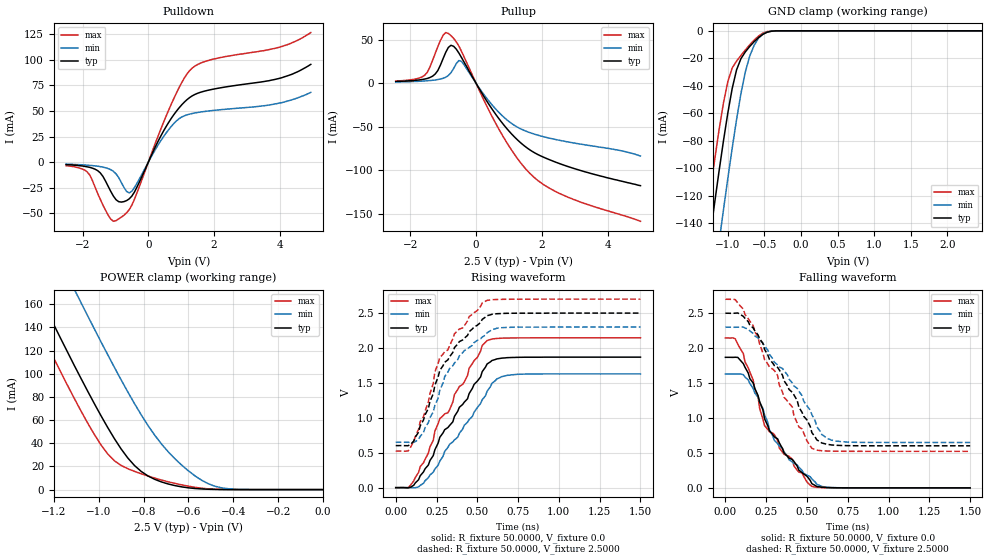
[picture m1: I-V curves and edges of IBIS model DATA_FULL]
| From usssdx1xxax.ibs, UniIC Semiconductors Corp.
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|   Model DATA_FULL
[Model]  DATA_FULL
Model_type   I/O
Polarity   Non-Inverting
Enable   Active-High
Vinl =   940.000mV
Vinh =   1.560V
Vmeas =   1.250V
Vref =   1.250V
Cref =   30.000pF
Rref =   50.000Ohm
C_comp   2.2640pF   2.2480pF   2.2810pF
[Temperature Range]   25.0000   0.1250k   -55.0000
[Voltage Range]   2.5000V   2.3000V   2.7000V
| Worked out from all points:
|   slope of the pulldown table from 0 to 0.375 V, typ, clamps not added: 14.9 ohm
|   slope of the pullup table from 0 to 0.375 V, typ, clamps not added: 16.1 ohm
|   GND clamp passes 1 mA (typ) near -0.46 V on its own axis
|   POWER clamp passes 1 mA (typ) near -0.57 V on its own axis
|   rising waveform, R_fixture 50.0000, V_fixture 0.0: 20-80 % time 280ps typ, 285ps min, 266ps max; typ from 0 V to 1.87 V
|   rising waveform, R_fixture 50.0000, V_fixture 2.5000: 20-80 % time 240ps typ, 219ps min, 234ps max; typ from 0.602 V to 2.5 V
|   falling waveform, R_fixture 50.0000, V_fixture 0.0: 20-80 % time 251ps typ, 242ps min, 261ps max; typ from 1.87 V to 0 V
|   falling waveform, R_fixture 50.0000, V_fixture 2.5000: 20-80 % time 282ps typ, 285ps min, 258ps max; typ from 2.5 V to 0.602 V
[Pulldown]
|Voltage   I(typ)   I(min)   I(max)
-2.5V     -2.3mA     -1.9mA     -3.4mA
-1.86V    -4.5mA     -2.9mA     -9.4mA
-1.46V    -10.4mA    -4.3mA     -36.1mA
-1.14V    -28.5mA    -7.3mA     -55.5mA
-980mV    -36.59mA   -11.4mA    -56.94mA
-660mV    -37.43mA   -28.47mA   -49.35mA
-500mV    -33.03mA   -28.27mA   -41.88mA
540mV     34.67mA    28.4mA     44.84mA
1.26V     63.12mA    46.94mA    89.43mA
1.9V      70.74mA    50.2mA     99.89mA
4.06V     82.4mA     58.1mA     112.8mA
4.94V     95.4mA     68.1mA     126.4mA
[Pullup]
|Voltage   I(typ)   I(min)   I(max)
-2.44V    1.9mA      1.4mA      2.4mA
-1.56V    4.7mA      2.5mA      9.1mA
-1.16V    14.5mA     4.2mA      41.88mA
-1V       28.2mA     5.6mA      55.08mA
-840mV    41.02mA    8.81mA     57.01mA
-680mV    42.28mA    16.81mA    51.38mA
-520mV    34.55mA    25.99mA    42.56mA
-440mV    29.38mA    24.95mA    36.47mA
680mV     -39.91mA   -32.96mA   -51.69mA
1.64V     -76.62mA   -56.8mA    -103.6mA
2.76V     -95.22mA   -67.18mA   -130.3mA
5V        -117.6mA   -83.6mA    -158.5mA
[GND_clamp]
|Voltage   I(typ)   I(min)   I(max)
-2.5V     -683.1mA   -736.1mA   -653.6mA
-1.3V     -173.1mA   -226.8mA   -141.1mA
-1.24V    -149mA     -202.4mA   -117.2mA
-1.18V    -125.4mA   -178.1mA   -94.12mA
-1.12V    -102.4mA   -154.2mA   -72.32mA
-1.06V    -80.41mA   -130.7mA   -52.79mA
-1V       -59.95mA   -107.7mA   -37.03mA
-880mV    -28.39mA   -64.58mA   -22.05mA
-760mV    -15.32mA   -29.84mA   -13.95mA
-700mV    -11.37mA   -18.38mA   -10.19mA
-520mV    -2.567mA   -2.292mA   -1.702mA
2.48V     19.82nA    1.016uA    2.464nA
[POWER_clamp]
|Voltage   I(typ)   I(min)   I(max)
-2.49V    671mA      736.6mA    644.5mA
-1.35V    201.6mA    268.3mA    172.7mA
-1.32V    189.6mA    256.3mA    160.6mA
-1.26V    165.8mA    232.4mA    136.8mA
-1.11V    107.6mA    173.4mA    79.15mA
-1.08V    96.37mA    161.8mA    68.24mA
-960mV    53.65mA    116.5mA    30.86mA
-840mV    20.7mA     74.06mA    15.7mA
-720mV    6.602mA    39.33mA    8.242mA
-600mV    1.533mA    16.16mA    2.964mA
-450mV    76.58uA    1.436mA    135uA
0V        21.05nA    42.84nA    5.083nA
[Ramp]
| variable   typ   min   max
dV/dt_r  1.1214/0.2791n   0.9774/0.2802n   1.2876/0.2672n
dV/dt_f  1.1387/0.2788n   0.9901/0.2809n   1.3062/0.2561n
R_load = 50.0000
[Rising Waveform]
R_fixture= 50.0000
V_fixture= 0.0
V_fixture_min= 0.0
V_fixture_max= 0.0
|time   V(typ)   V(min)   V(max)
0s        0V         0V         0V
75.76ps   -3.298mV   323.4uV    -359.3uV
170ps     224.4mV    61.95mV    355.9mV
270ps     720.7mV    379.7mV    988.1mV
320ps     861mV      576.4mV    1.073V
360ps     1.021V     683.7mV    1.333V
560ps     1.771V     1.381V     2.107V
620ps     1.844V     1.558V     2.137V
710ps     1.864V     1.616V     2.144V
1.5ns     1.869V     1.629V     2.146V
[Rising Waveform]
R_fixture= 50.0000
V_fixture= 2.5000
V_fixture_min= 2.3000
V_fixture_max= 2.7000
|time   V(typ)   V(min)   V(max)
0s        602.1mV    649.9mV    523mV
75.76ps   600.5mV    649.2mV    525.9mV
140ps     795.1mV    690.5mV    838.2mV
230ps     1.345V     1.084V     1.491V
240ps     1.467V     1.178V     1.659V
270ps     1.679V     1.392V     1.862V
390ps     2.092V     1.888V     2.271V
530ps     2.41V      2.156V     2.646V
650ps     2.495V     2.291V     2.697V
1.5ns     2.5V       2.3V       2.7V
[Falling Waveform]
R_fixture= 50.0000
V_fixture= 0.0
V_fixture_min= 0.0
V_fixture_max= 0.0
|time   V(typ)   V(min)   V(max)
0s        1.869V     1.629V     2.146V
60.61ps   1.87V      1.629V     2.133V
140ps     1.644V     1.546V     1.716V
200ps     1.323V     1.299V     1.304V
240ps     988.9mV    1.045V     891.6mV
300ps     729.1mV    679.5mV    762.9mV
330ps     646.2mV    600.4mV    571.8mV
530ps     59.69mV    126.8mV    20.18mV
650ps     2.335mV    4.513mV    1.058mV
1.5ns     0V         -1.833uV   0V
[Falling Waveform]
R_fixture= 50.0000
V_fixture= 2.5000
V_fixture_min= 2.3000
V_fixture_max= 2.7000
|time   V(typ)   V(min)   V(max)
0s        2.5V       2.3V       2.7V
60.61ps   2.501V     2.299V     2.694V
170ps     2.291V     2.212V     2.324V
240ps     1.982V     2.026V     1.838V
320ps     1.725V     1.76V      1.609V
360ps     1.531V     1.675V     1.295V
530ps     790.5mV    1.047V     565.9mV
590ps     643.1mV    765.1mV    531.2mV
680ps     609.2mV    668.8mV    524.6mV
1.5ns     602.1mV    649.9mV    523mV
